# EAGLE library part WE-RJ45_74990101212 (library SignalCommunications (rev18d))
WE-RJ45 LAN Transformer Order Code 74990101212 Design THT xBase-T 10/100 Base-T Ports 1x1 Application Standard Tab Position UP LED (Left-Right) GREEN-YELLOW EMI Fingers No Details see: http://katalog.we-online.de/en/pbs/WE-LAN-RJ45 Created by Yingchun Shan 2016 (C) Wurth Elektronik
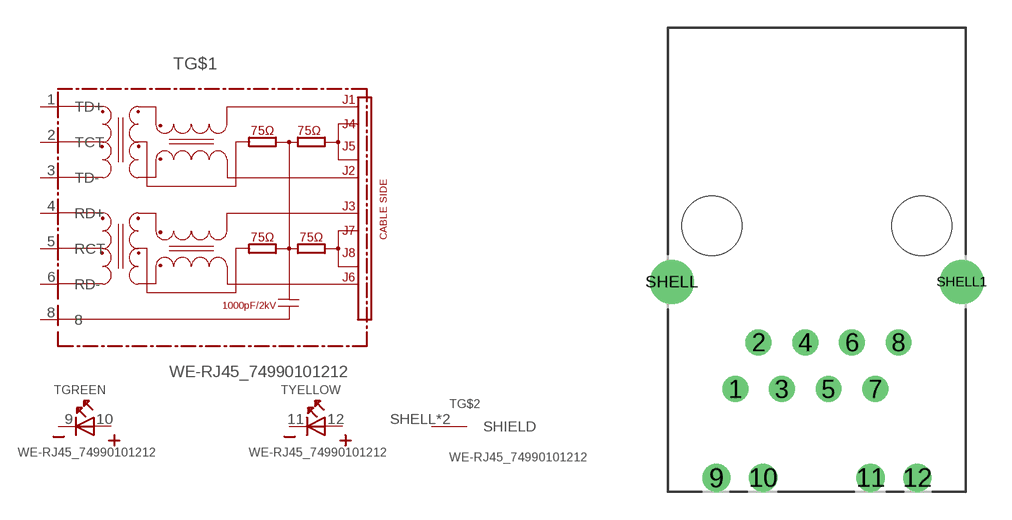
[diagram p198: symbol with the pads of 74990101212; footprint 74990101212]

Designator prefix T; gates G$1=74990101212 GREEN=LED_2PIN YELLOW=LED_2PIN G$2=SHIELD

## WE-RJ45_74990101212  [74990101212]
1  G$1:TD+
2  G$1:TCT
3  G$1:TD-
4  G$1:RD+
5  G$1:RCT
6  G$1:RD-
8  G$1:8
9  GREEN:K  pas
10  GREEN:A  pas
11  YELLOW:K  pas
12  YELLOW:A  pas
SHELL  G$2:SHIELD  pas
SHELL1  G$2:SHIELD  pas

## Footprint 74990101212 (pad centres in mm)
drill 0.9: 1 -4.445,-5.84; 2 -3.175,-3.3; 3 -1.905,-5.84; 4 -0.635,-3.3; 5 0.635,-5.84; 6 1.905,-3.3; 7 3.175,-5.84; 8 4.445,-3.3
drill 1.02: 9 -5.465,-10.67; 10 -2.925,-10.67; 11 2.925,-10.67; 12 5.465,-10.67
drill 1.6: SHELL -7.9,0; SHELL1 7.9,0
hole 3.25 at -5.715,3.05
hole 3.25 at 5.715,3.05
